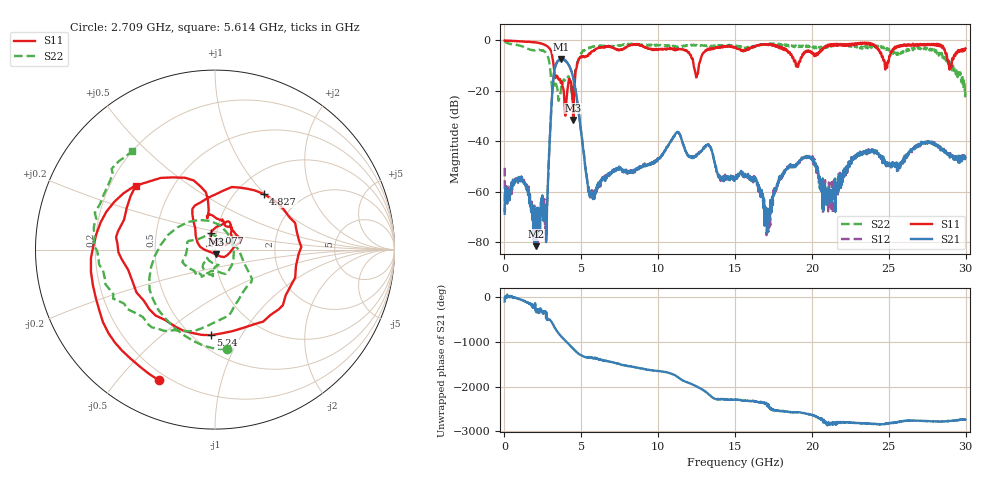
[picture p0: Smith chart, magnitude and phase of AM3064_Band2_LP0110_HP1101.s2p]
# Hz S DB R 50.0
!freq dBS11 angS11 dBS21 angS21 dBS12 angS12 dBS22 angS22
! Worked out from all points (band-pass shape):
!   1600 points, 10 MHz to 29.98 GHz, reference 50 ohm
!   highest |S21| = -7.42 dB at 3.703 GHz (marker M1); lowest = -81.5 dB at 2.053 GHz (marker M2)
!   |S21| within 3 dB of the highest: 3.306 GHz to 4.238 GHz (931.6 MHz wide, 24.7 % of centre)
!   lowest |S11| = -31.5 dB at 4.471 GHz (marker M3), VSWR 1.05, Z = 50.5 - j2.63 ohm
!   |S11| at or under -10 dB: 3.2 GHz to 4.719 GHz (1.519 GHz wide, 38.4 % of centre); 12.31 GHz to 12.64 GHz (332.8 MHz wide, 2.67 % of centre); 28.91 GHz to 29.08 GHz (163.9 MHz wide, 0.565 % of centre)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
!   |S22| runs from -23.9 to -0.3 dB; largest |S21 - S12| = 0.015
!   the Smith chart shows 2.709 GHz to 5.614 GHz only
!   S11 on the Smith chart (normalised r, x): 2.709 GHz: 0.17, -0.64; 4.077 GHz: 0.94, +0.18; 4.827 GHz: 1.32, +0.99; 5.24 GHz: 0.61, -0.75; 5.614 GHz: 0.31, +0.32
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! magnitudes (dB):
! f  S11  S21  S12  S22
! 10 MHz  0.0  -68.7  -50.4  -0.3
! 1.06 GHz  -0.4  -54.4  -54.4  -2.2
! 2.053 GHz  -0.8  -81.5  -71.4  -3.8
! 2.709 GHz  -2.0  -79.9  -70.1  -5.1
! 3.196 GHz  -9.8  -14.4  -14.2  -16.6
! 3.703 GHz  -16.2  -7.4  -7.4  -17.6
! 4.077 GHz  -20.4  -8.8  -8.7  -15.0
! 4.471 GHz  -31.5  -14.8  -14.6  -21.7
! 4.827 GHz  -7.7  -28.4  -28.3  -7.0
! 5.015 GHz  -6.7  -37.8  -37.5  -5.2
! 5.24 GHz  -6.4  -48.9  -48.9  -3.7
! 5.614 GHz  -4.9  -61.1  -59.8  -2.9
! 10 GHz  -3.6  -47.1  -46.9  -1.9
! 11.27 GHz  -3.5  -36.4  -36.3  -2.7
! 15 GHz  -2.7  -54.4  -54.3  -2.0
! 17.14 GHz  -1.8  -70.5  -71.2  -1.4
! 18.3 GHz  -3.3  -51.1  -51.2  -2.2
! 19.99 GHz  -4.6  -46.6  -46.6  -2.2
! 20.82 GHz  -2.7  -60.6  -65.1  -2.4
! 23.01 GHz  -1.4  -45.1  -45.5  -2.6
! 25 GHz  -8.2  -49.1  -48.7  -3.3
! 29.98 GHz  -3.2  -46.4  -46.6  -20.3
